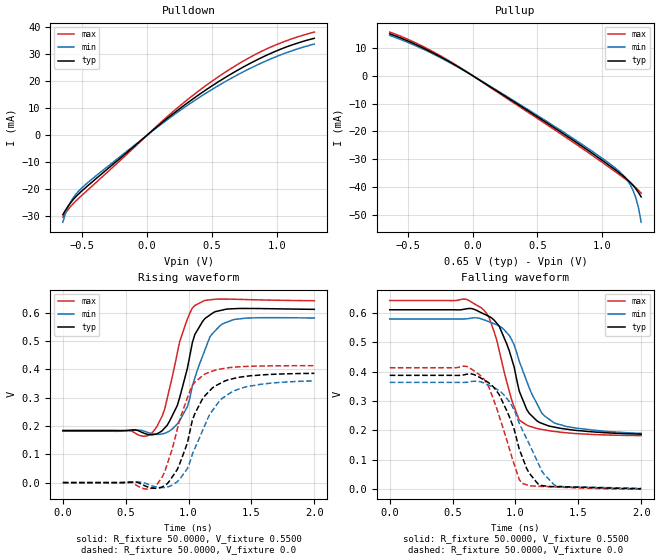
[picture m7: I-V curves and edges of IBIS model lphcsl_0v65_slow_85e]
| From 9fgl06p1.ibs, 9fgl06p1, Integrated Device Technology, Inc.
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[Model]   lphcsl_0v65_slow_85e
Model_type Output
Polarity   Inverting
Enable   Active-High
Vmeas =  0.4000V
Cref =   2.0000pF
Rref =   0.0
Vref =   0.4000V
C_comp   1.1000pF   1.0000pF   1.2000pF
[Temperature Range]   25.0000   85.0000   -40.0000
[Voltage Range]   0.6500V   0.6200V   0.6800V
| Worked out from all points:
|   slope of the pulldown table from 0 to 0.098 V, typ, clamps not added: 24.6 ohm
|   slope of the pullup table from 0 to 0.098 V, typ, clamps not added: 34 ohm
|   rising waveform, R_fixture 50.0000, V_fixture 0.5500: 20-80 % time 147ps typ, 175ps min, 152ps max; typ from 0.184 V to 0.612 V
|   rising waveform, R_fixture 50.0000, V_fixture 0.0: 20-80 % time 195ps typ, 234ps min, 174ps max; typ from 0 V to 0.386 V
|   falling waveform, R_fixture 50.0000, V_fixture 0.5500: 20-80 % time 190ps typ, 221ps min, 177ps max; typ from 0.61 V to 0.187 V
|   falling waveform, R_fixture 50.0000, V_fixture 0.0: 20-80 % time 198ps typ, 234ps min, 188ps max; typ from 0.387 V to 0.002 V
[Pulldown]
|Voltage   I(typ)   I(min)   I(max)
-650mV    -29.53mA   -32.32mA   -30.49mA
-630mV    -27.88mA   -29.08mA   -28.98mA
-590mV    -25.09mA   -24.79mA   -26.48mA
-550mV    -22.86mA   -21.99mA   -24.47mA
-510mV    -20.99mA   -19.89mA   -22.65mA
-370mV    -15.18mA   -14.16mA   -16.53mA
10mV      415.6uA    382.9uA    460.3uA
230mV     9.045mA    8.358mA    9.971mA
510mV     18.6mA     17.25mA    20.36mA
770mV     26.03mA    24.22mA    28.28mA
1.01V     31.54mA    29.44mA    33.86mA
1.29V     35.98mA    33.84mA    38.29mA
[Pullup]
|Voltage   I(typ)   I(min)   I(max)
-640mV    15.06mA    14.49mA    15.68mA
-520mV    12.87mA    12.35mA    13.49mA
-360mV    9.457mA    9.049mA    9.963mA
-60mV     1.732mA    1.649mA    1.841mA
600mV     -17.81mA   -17.25mA   -18.45mA
1.06V     -32.46mA   -31.73mA   -33.16mA
1.16V     -35.99mA   -35.72mA   -36.56mA
1.22V     -38.54mA   -39.59mA   -38.7mA
1.24V     -39.57mA   -41.53mA   -39.46mA
1.26V     -40.75mA   -44.1mA    -40.29mA
1.28V     -42.07mA   -47.64mA   -41.21mA
1.3V      -43.57mA   -52.66mA   -42.27mA
[Ramp]
| variable   typ   min   max
dV/dt_r  0.2315/0.2154n   0.2156/0.2436n   0.2477/0.1882n
dV/dt_f  0.2565/0.2195n   0.2357/0.2462n   0.2789/0.1861n
R_load = 50.0000
[Rising Waveform]
R_fixture= 50.0000
V_fixture= 0.5500
V_fixture_min= 0.5200
V_fixture_max= 0.5800
|time   V(typ)   V(min)   V(max)
0s        184mV      183.2mV    181.4mV
710ps     168.7mV    172.6mV    176.2mV
810ps     192.9mV    173.9mV    259.7mV
910ps     271.8mV    207.1mV    456.7mV
990ps     402.6mV    267.9mV    577.3mV
1.05ns    523.3mV    369.5mV    625.5mV
1.17ns    592mV      514.8mV    645.6mV
1.27ns    609.5mV    560.6mV    648.1mV
1.47ns    614.9mV    581.2mV    646.3mV
2ns       611.9mV    581.3mV    642.3mV
[Rising Waveform]
R_fixture= 50.0000
V_fixture= 0.0
V_fixture_min= 0.0
V_fixture_max= 0.0
|time   V(typ)   V(min)   V(max)
0s        0V         0V         0V
670ps     -14.54mV   -4.773mV   -23.2mV
790ps     -15.5mV    -17.61mV   19.6mV
910ps     45.95mV    3.042mV    188.2mV
990ps     139.2mV    49.18mV    299.1mV
1.03ns    220.5mV    100.9mV    343.7mV
1.13ns    306.9mV    203.1mV    383.7mV
1.25ns    350mV      291mV      400.9mV
1.37ns    368.8mV    325.7mV    407.8mV
2ns       385.8mV    359.4mV    412.9mV
[Falling Waveform]
R_fixture= 50.0000
V_fixture= 0.5500
V_fixture_min= 0.5200
V_fixture_max= 0.5800
|time   V(typ)   V(min)   V(max)
0s        609.5mV    578.3mV    640.9mV
610ps     612.8mV    578.6mV    645mV
750ps     595mV      575.5mV    608mV
870ps     554.4mV    554.2mV    472.3mV
990ps     414.7mV    490.1mV    279.5mV
1.03ns    333.6mV    435.1mV    235.6mV
1.09ns    270.9mV    366.8mV    218.1mV
1.21ns    224mV      258.6mV    203.3mV
1.31ns    211.3mV    225mV      196.6mV
2ns       187.4mV    190mV      182.5mV
[Falling Waveform]
R_fixture= 50.0000
V_fixture= 0.0
V_fixture_min= 0.0
V_fixture_max= 0.0
|time   V(typ)   V(min)   V(max)
0s        387mV      363mV      412.8mV
610ps     390.5mV    363.3mV    417.5mV
730ps     376.5mV    364mV      383.1mV
790ps     360.9mV    353.2mV    345.5mV
870ps     322.2mV    334.7mV    249.6mV
970ps     225.8mV    285.2mV    111.5mV
1.05ns    114.6mV    206.5mV    21.02mV
1.19ns    14.03mV    80.57mV    10.27mV
1.31ns    9.231mV    14.61mV    8.511mV
2ns       2.174mV    3.57mV     724.5uV
